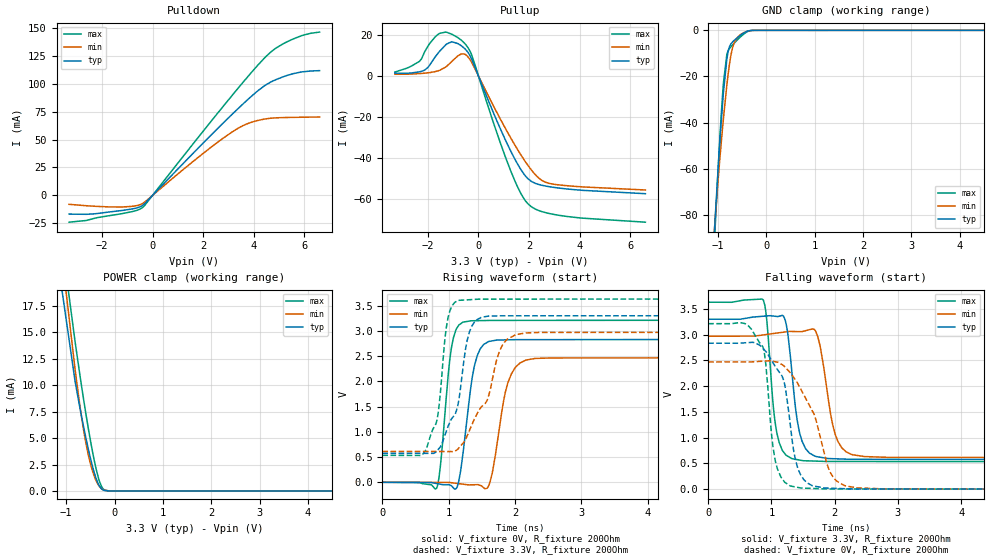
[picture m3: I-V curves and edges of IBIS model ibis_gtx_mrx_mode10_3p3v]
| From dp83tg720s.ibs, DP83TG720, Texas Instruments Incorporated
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| ibis_gtx_mrx_mode10_3p3v
[Model]   ibis_gtx_mrx_mode10_3p3v
Model_type   I/O
Polarity   Non-Inverting
Enable   Active-Low
Vinl = 0.99
Vinh = 2.31
Vmeas = 1.65
Vref = 1.65
Cref = 2pF
Rref = 100000
|   typ   min   max
C_comp   2.9pF   2.87pF   2.94pF
[Voltage Range]   3.3   2.97   3.63
[Temperature Range]   27   150   -40
[Pullup Reference]   3.3   2.97   3.63
[Pulldown Reference]   0   0   0
[Power Clamp Reference]   3.3   2.97   3.63
[GND Clamp Reference]   0   0   0
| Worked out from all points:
|   slope of the pulldown table from 0 to 0.495 V, typ, clamps not added: 42.2 ohm
|   slope of the pullup table from 0 to 0.495 V, typ, clamps not added: 32.8 ohm
|   GND clamp passes 1 mA (typ) near -0.45 V on its own axis
|   POWER clamp passes 1 mA (typ) near -0.37 V on its own axis
|   falling waveform, V_fixture 3.3V, R_fixture 200Ohm: 20-80 % time 157ps typ, 195ps min, 132ps max; typ from 3.3 V to 0.575 V
|   rising waveform, V_fixture 0V, R_fixture 200Ohm: 20-80 % time 167ps typ, 195ps min, 133ps max; typ from 0 V to 2.83 V
|   rising waveform, V_fixture 3.3V, R_fixture 200Ohm: 20-80 % time 277ps typ, 410ps min, 153ps max; typ from 0.575 V to 3.3 V
|   falling waveform, V_fixture 0V, R_fixture 200Ohm: 20-80 % time 254ps typ, 429ps min, 151ps max; typ from 2.83 V to 0 V
[Pulldown]
|   Voltage   I(typ)   I(min)   I(max)
-3.3V     -16.77mA   -7.996mA   -24.01mA
-2.32V    -16.56mA   -9.689mA   -20.66mA
-1.211V   -13.53mA   -10.42mA   -16.37mA
-676.5mV  -11.5mA    -9.369mA   -13.77mA
-399.3mV  -9.041mA   -7.33mA    -10.9mA
2.234V    52.23mA    41.75mA    64.12mA
3.046V    70.46mA    55.28mA    86.81mA
3.59V     82.23mA    62.68mA    101.7mA
4.412V    98.01mA    68.33mA    122.8mA
4.887V    103.8mA    69.47mA    132.1mA
5.877V    110.5mA    70mA       143mA
6.6V      111.8mA    70.21mA    146.3mA
[GND Clamp]
|   Voltage   I(typ)   I(min)   I(max)
-3.3V     -1.011A    -865.8mA   -1.126A
-1.082V   -91.37mA   -89.71mA   -96.69mA
-1.053V   -80.45mA   -81.02mA   -84.12mA
-963.6mV  -49.69mA   -56.87mA   -48.48mA
-894.3mV  -29.4mA    -40.34mA   -25.48mA
-815.1mV  -12.66mA   -23.94mA   -10.6mA
-765.6mV  -7.479mA   -15.54mA   -8.067mA
-726mV    -5.787mA   -10.39mA   -7.032mA
-676.5mV  -4.645mA   -6.247mA   -5.893mA
-567.6mV  -2.701mA   -2.49mA    -3.55mA
-419.1mV  -641.7uA   -597.9uA   -944.7uA
6.6V      0A         0A         0A
[Pullup]
|   Voltage   I(typ)   I(min)   I(max)
-3.3V     1.293mA    748.4uA    1.811mA
-2.33V    1.941mA    1.084mA    7.036mA
-2.142V   2.672mA    1.267mA    11.2mA
-1.538V   11.87mA    2.646mA    20.62mA
-1.053V   16.6mA     6.952mA    20.28mA
-815.1mV  15.72mA    9.702mA    18.66mA
-537.9mV  13.21mA    10.52mA    15.72mA
-280.5mV  8.592mA    6.897mA    10.64mA
1.125V    -32.76mA   -26.9mA    -41.43mA
1.957V    -50.09mA   -43.61mA   -62.32mA
2.788V    -53.99mA   -52.36mA   -67.04mA
6.6V      -57.42mA   -55.62mA   -71.3mA
[POWER Clamp]
|   Voltage   I(typ)   I(min)   I(max)
-3.3V     317.9mA    237mA      400.5mA
-1.181V   21.99mA    25.93mA    26.78mA
-815.1mV  10.35mA    11.45mA    14.1mA
-656.7mV  6.45mA     6.234mA    9.162mA
-587.4mV  4.9mA      4.403mA    7.158mA
-528mV    3.668mA    3.117mA    5.537mA
-458.7mV  2.373mA    1.935mA    3.791mA
-369.6mV  1.032mA    856.8uA    1.866mA
-310.2mV  435.4uA    402.4uA    888uA
-231mV    77.4uA     103.3uA    169.6uA
-62.7mV   288.7nA    1.815uA    282.8nA
6.6V      0A         0A         0A
[Ramp]
R_load = 200
|   typ   min   max
dV/dt_r   1.69835/1.65597e-10   1.48038/1.94504e-10   1.92667/1.31892e-10
dV/dt_f   1.63524/1.56652e-10   1.41531/1.94264e-10   1.85752/1.31232e-10
[Falling Waveform]
V_fixture = 3.3V
V_fixture_min = 2.97V
V_fixture_max = 3.63V
R_fixture = 200Ohm
C_fixture = 0F
|   Time   V(typ)   V(min)   V(max)
0s        3.3V       2.97V      3.63V
871.3ps   3.358V     2.995V     3.673V
1.078ns   3.354V     3.03V      1.143V
1.217ns   3.282V     3.053V     681.3mV
1.317ns   2.362V     3.062V     597.1mV
1.54ns    786.2mV    3.078V     550.8mV
1.732ns   628mV      2.963V     543.5mV
2.003ns   590.3mV    1.089V     537.9mV
2.264ns   579.6mV    675.8mV    537.6mV
6ns       574.7mV    611.2mV    534.2mV
[Rising Waveform]
V_fixture = 0V
V_fixture_min = 0V
V_fixture_max = 0V
R_fixture = 200Ohm
C_fixture = 0F
|   Time   V(typ)   V(min)   V(max)
0s        1.562uV    20.75uV    660.8nV
818ps     -24.53mV   -2.725mV   -119.1mV
1.037ns   -66.9mV    -7.809mV   2.633V
1.129ns   -84.8mV    -23.11mV   3.067V
1.214ns   558.2mV    -37.23mV   3.172V
1.387ns   2.304V     -48.49mV   3.201V
1.6ns     2.789V     -74.64mV   3.206V
1.887ns   2.823V     1.951V     3.208V
2.166ns   2.826V     2.422V     3.208V
6ns       2.831V     2.467V     3.211V
[Rising Waveform]
V_fixture = 3.3V
V_fixture_min = 2.97V
V_fixture_max = 3.63V
R_fixture = 200Ohm
C_fixture = 0F
|   Time   V(typ)   V(min)   V(max)
0s        574.7mV    611.2mV    534.2mV
659.6ps   573.5mV    609.9mV    647mV
835.4ps   641mV      609.6mV    1.324V
989ps     1.104V     609.3mV    3.256V
1.139ns   1.534V     659.8mV    3.602V
1.277ns   2.803V     918.1mV    3.614V
1.381ns   3.163V     1.237V     3.623V
1.792ns   3.299V     2.675V     3.629V
2.01ns    3.299V     2.923V     3.629V
6ns       3.3V       2.97V      3.63V
[Falling Waveform]
|Gnd
V_fixture = 0V
V_fixture_min = 0V
V_fixture_max = 0V
R_fixture = 200Ohm
C_fixture = 0F
|   Time   V(typ)   V(min)   V(max)
0s        2.834V     2.47V      3.214V
861.9ps   2.737V     2.485V     2.769V
1.053ns   2.399V     2.476V     603.8mV
1.195ns   2.11V      2.398V     160.1mV
1.287ns   1.366V     2.275V     69.26mV
1.378ns   580.6mV    2.125V     43.53mV
1.509ns   189.6mV    1.837V     19.85mV
1.934ns   18.56mV    318.3mV    4.238mV
2.158ns   9.132mV    67.64mV    4.005mV
6ns       1.55uV     20.79uV    849.3nV
